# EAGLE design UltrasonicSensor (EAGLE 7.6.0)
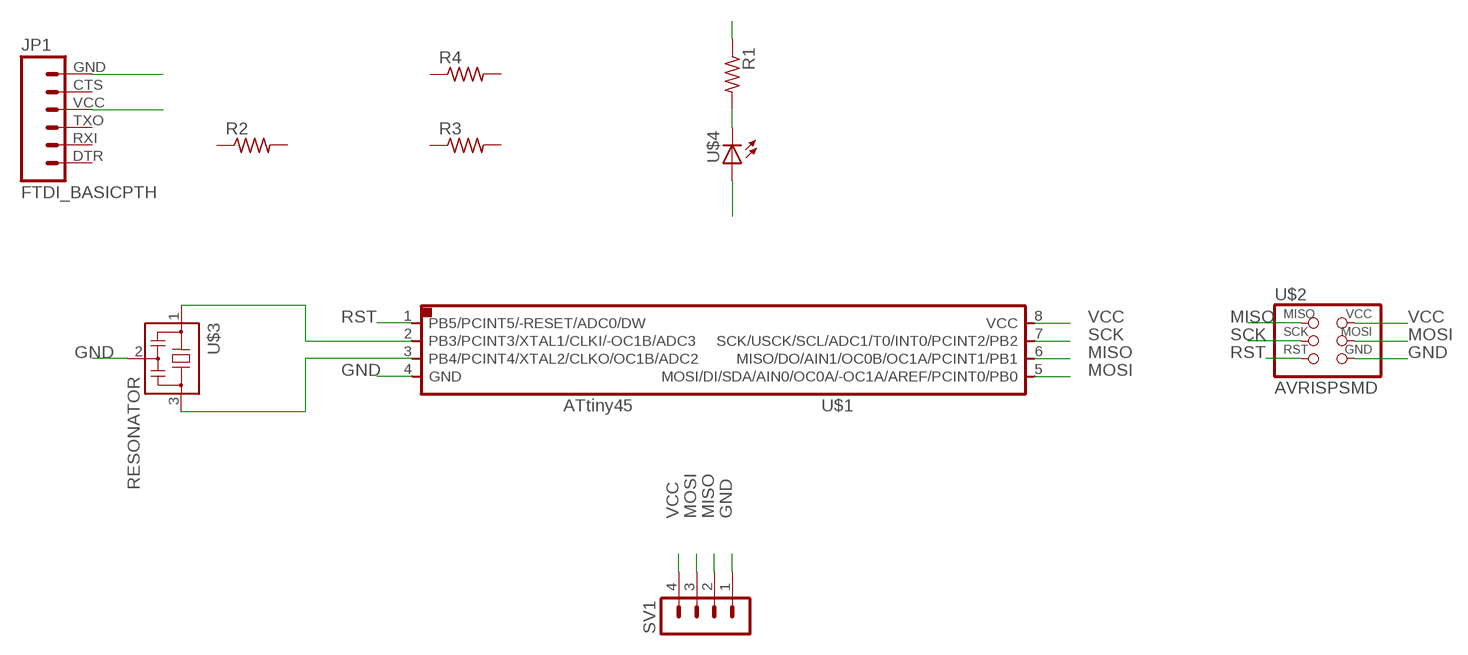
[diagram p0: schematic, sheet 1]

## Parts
JP1  FTDI_BASICPTH  [FTDI_BASIC]
R1  RES-US1206FAB  [R1206FAB]
R2  RES-US1206FAB  [R1206FAB]
R3  RES-US1206FAB  [R1206FAB]
R4  RES-US1206FAB  [R1206FAB]
SV1  MA04-1  [MA04-1]
U$1  ATTINY45SI  [SOIC8]
U$2  AVRISPSMD  [2X03SMD]
U$3  RESONATOR  [EFOBM]
U$4  LED5MM  [5MM]

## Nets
GND: JP1.GND R1.1 SV1.1 U$1.4(GND) U$2.6(GND) U$3.2
MISO: SV1.2 U$1.6(MISO/DO/AIN1/OC0B/OC1A/PCINT1/PB1) U$2.1(MISO)
MOSI: SV1.3 U$1.5(MOSI/DI/SDA/AIN0/OC0A/-OC1A/AREF/PCINT0/PB0) U$2.4(MOSI)
N$1: R1.2 U$4.OUT(C)
N$12: U$1.2(PB3/PCINT3/XTAL1/CLKI/-OC1B/ADC3) U$3.1
N$13: U$1.3(PB4/PCINT4/XTAL2/CLKO/OC1B/ADC2) U$3.3
RST: U$1.1(PB5/PCINT5/-RESET/ADC0/DW) U$2.5(RST)
SCK: U$1.7(SCK/USCK/SCL/ADC1/T0/INT0/PCINT2/PB2) U$2.3(SCK) U$4.IN(A)
VCC: JP1.VCC SV1.4 U$1.8(VCC) U$2.2(VCC)
Unconnected: JP1.CTS JP1.DTR JP1.RXI JP1.TXO R2.1 R2.2 R3.1 R3.2 R4.1 R4.2

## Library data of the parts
JP1 = SparkFun:FTDI_BASIC: FTDI Basic: 3.3V and 5V
R1-R4 = fab:RES-US: Resistor (US Symbol)
SV1 = con-lstb:MA04-1: PIN HEADER; OC_FARNELL: unknown; OC_NEWARK: unknown
U$1 = fab:ATTINY45
U$2 = fab:AVRISP
U$3 = fab:RESONATOR
U$4 = FabLab:LED

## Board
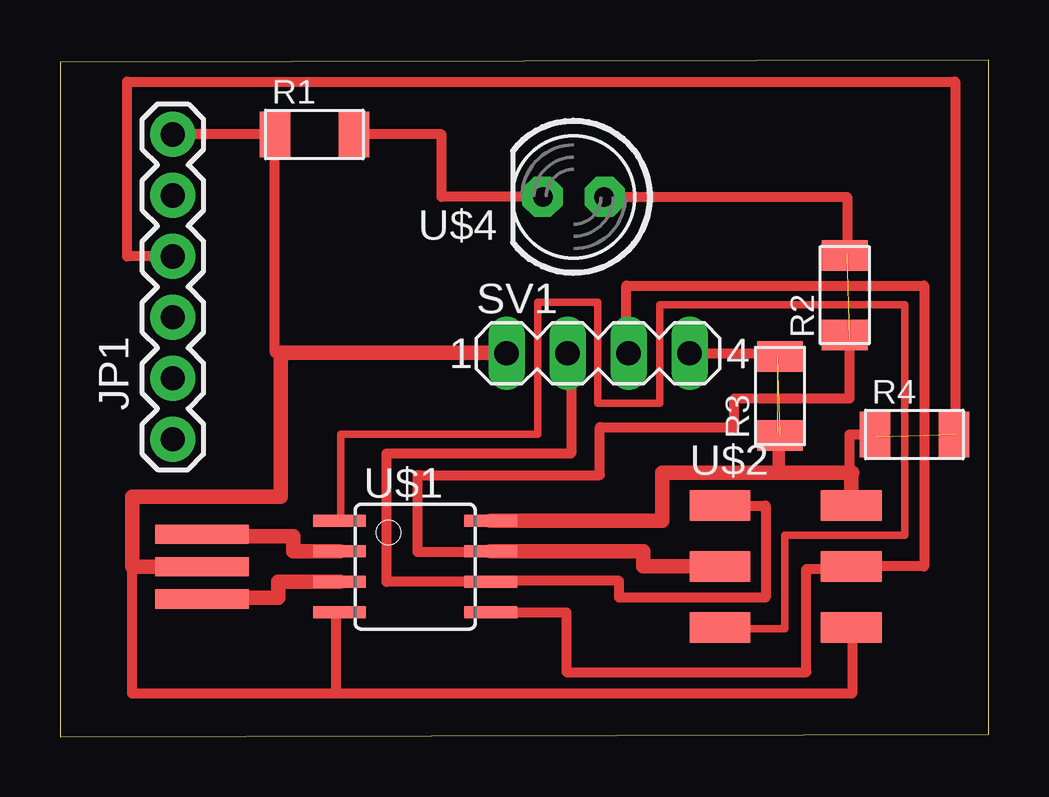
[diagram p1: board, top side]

Size 38.7 x 28.2 mm. Coordinates in mm from the lower left corner, seen from the top.
Outline: 0,0 38.7,0.1 38.7,28.2 0,28.1 0,0
Copper layers (1*16): Top 0.035mm / dielectric 1.5mm / Bottom 0.035mm
Design rules "default": minimum track width 10mil, minimum drill 24mil, track to track 8mil, track to pad 8mil, pad to pad 8mil, via to via 8mil, smd to smd 8mil, copper to edge 40mil, drill to drill 8mil, minimum pad ring 10mil, minimum via ring 8mil, stop-mask expansion 4mil, vias tented up to drill 0mil, thermal gap 10mil

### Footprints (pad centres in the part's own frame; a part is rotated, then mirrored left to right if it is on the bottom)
FTDI_BASIC = drill 1.016 pad 1.88: CTS 10.16,0; DTR 0,0; GND 12.7,0; RXI 2.54,0; TXO 5.08,0; VCC 7.62,0
R1206FAB = smd 1.27 x 1.905: 1 -1.651,0; 2 1.651,0
MA04-1 = drill 1.016 long: 1 -3.81,0; 2 -1.27,0; 3 1.27,0; 4 3.81,0
SOIC8 = smd 0.5 x 2.2: 1 -1.905,-3.154; 2 -0.645,-3.154; 3 0.625,-3.154; 4 1.895,-3.154; 5 1.905,3.154; 6 0.635,3.154; 7 -0.635,3.154; 8 -1.905,3.154
2X03SMD = smd 2.54 x 1.27: 1 -2.54,2.54; 2 2.92,2.54; 3 -2.54,0; 4 2.92,0; 5 -2.54,-2.54; 6 2.92,-2.54
EFOBM = smd 0.8 x 3.9: 1 -1.35,0; 2 0,0; 3 1.35,0
5MM = drill 0.813 pad 1.422: IN -1.27,0; OUT 1.27,0

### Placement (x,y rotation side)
JP1  4.7,12.4 90 top
R1  10.6,25.1 0 top
R2  32.7,18.4 90 top
R3  30,14.2 90 top
R4  35.6,12.6 0 top
SV1  22.42,15.98 0 top
U$1  14.8,7.09 270 top
U$2  30.04,7.09 0 top
U$3  5.91,7.09 270 top
U$4  21.4,22.5 180 top

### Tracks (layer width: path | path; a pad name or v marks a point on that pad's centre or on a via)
GND
  Top 0.406: U$2.6 33,4.55 33,1.8 11.5,1.8 | 11.5,1.8 3,1.8 3,7.09 | U$1.4 11.5,5.2 11.5,1.8 | JP1.GND R1.1 8.95,16 9.2,16
  Top 0.61: U$3.2 3,7.09 3,10 9.2,10 9.2,16 18.61,16 SV1.1
MISO
  Top 0.406: U$2.1 29.4,9.63 29.4,5.8 23.3,5.8 23.3,6.5 17.95,6.5 U$1.6 13.6,6.45 13.6,11.8 21.3,11.8 21.3,15.98 SV1.2
MOSI
  Top 0.406: U$1.5 21.1,5.18 21.1,2.7 31.1,2.7 31.1,7 32.96,7 U$2.4 36,7.1 36,18.8 23.6,18.8 23.6,15.98 SV1.3
N$1  (via drill 0.6 pad 1.68)
  Top 0.406: U$4.OUT v20.1,22.5 15.9,22.5 15.9,25.1 R1.2
N$12
  Top 0.61: U$1.2 9.72,7.73 9.72,8.36 5.91,8.36 U$3.1
N$13
  Top 0.61: U$1.3 9.1,6.46 9.1,5.8 5.91,5.8 U$3.3
RST
  Top 0.305: U$1.1 11.7,9 11.7,12.6 19.9,12.6 19.9,18.1 22.4,18.1 22.4,13.9 25,13.9 25,18 35.2,18 35.2,8.4 30.2,8.4 30.2,4.5 27.5,4.5 U$2.5
SCK  (via drill 0.6 pad 1.68)  (1 unrouted)
  Top 0.406: U$4.IN v22.7,22.5 32.8,22.5 32.8,20.1 | U$2.3 24.3,7.09 24.3,7.7 14.9,7.7 14.9,10.9 22.5,10.9 22.5,12.9 28.1,12.9 28.1,14.1 32.9,14.1 32.9,16.6
  Top 0.61: U$1.7 24.3,7.73 24.3,7.7 24.3,7.1 U$2.3
VCC  (3 unrouted)
  Top 0.406: SV1.4 29.9,15.98 29.9,15.8 | 30,11 29.9,11 29.9,12.7 | 30,11 30,12.6 | 32.9,11 30,11 | JP1.VCC 2.8,20.02 2.8,27.3 37.3,27.3 37.3,12.6 | 33,11 32.9,11 | 32.9,11 32.9,12.6 34,12.6 34,12.5
  Top 0.61: U$1.8 25.1,9 25.1,11 29.9,11 32.96,11 | 33,11 32.96,11 | 32.96,11 U$2.2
